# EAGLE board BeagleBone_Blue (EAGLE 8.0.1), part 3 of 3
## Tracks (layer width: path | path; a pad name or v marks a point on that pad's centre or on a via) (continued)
UART5_RX  (via drill 0.25 pad 0.46)
  Top 0.152: v68.38,34.29 68.73,34.29 69.01,34.57 70.46,34.57 71.04,33.98 71.04,26.36 70.31,25.63 68.15,25.63 67.06,24.54 67.06,22 67.51,21.54 69.42,21.54 v69.7,21.26 | 73.03,8.87 UT5.3 73,10.13 72.69,10.44 v69.7,10.44 | SIP.U2 62.31,37.52 v62.03,37.52
  Bottom 0.152: R131.2 63.32,32.51 63.5,32.69 65.48,32.69 65.84,33.05 65.84,34.24 | 65.84,34.49 65.35,34.98 64.06,34.98 63.88,35.15 63.88,35.94 63.7,36.12 62.99,36.12 62.79,36.32 62.79,37.03 62.31,37.52 v62.03,37.52 | 65.84,34.49 66.09,34.49 | 66.09,34.49 67.84,34.49 68.05,34.29 v68.38,34.29 | 65.84,34.49 65.84,34.24 | v69.7,21.26 v69.7,10.44 | 65.84,34.24 66.09,34.49
UART5_TX  (via drill 0.25 pad 0.46)
  Top 0.152: SIP.U1 63.42,36.75 62.97,36.75 62.76,36.55 62.31,36.55 v62.03,36.83 | v65.89,16.41 66.19,16.41 66.85,15.75 66.85,12.95 68.12,11.68 68.12,11.12 69.29,9.96 71.81,9.96 72.01,9.75 UT5.4
  Bottom 0.152: v65.89,16.41 66.06,16.59 66.06,20.22 65.05,21.23 65.05,22.63 56.01,31.67 53.29,31.67 51.77,33.2 51.77,33.68 52.05,33.96 56.9,33.96 58.73,35.79 59.64,35.79 60.07,35.36 60.07,35.1 60.35,34.82 60.86,34.82 61.21,35.18 61.21,35.59 60.27,36.52 60.27,36.93 60.55,37.21 61.65,37.21 v62.03,36.83 62.48,36.37 62.48,36.14 62.94,35.69 63.2,35.69 R129.2
USB0_D_N  (via drill 0.25 pad 0.46)
  Top 0.152: U3.2 8.03,39.57 7.49,39.04 6.88,39.04 6.48,38.63 v6.48,38.48 6.88,38.08 7.39,38.08 9.22,39.9 v9.73,39.9 | SIP.N18 41.96,31.8 v41.68,31.8
  Route2 0.152: v41.68,31.8 40.89,31.8 40.51,31.42 31.93,31.42 29.87,33.48 29.87,35.43 28.88,36.42 v27.79,36.42
  Bottom 0.152: X4.D- 5.7,37.7 v6.48,38.48 | v9.73,39.9 11.25,41.43 24.59,41.43 25.09,40.92 25.09,39.34 25.27,39.17 25.53,39.17 25.7,39.34 25.7,39.7 25.88,39.88 26.14,39.88 26.34,39.67 26.34,37.29 27.2,36.42 v27.79,36.42
USB0_D_P  (via drill 0.25 pad 0.46)
  Top 0.152: U3.1 7.53,39.58 7.29,39.34 6.76,39.34 6.4,38.99 6.17,38.99 v5.69,38.51 6.43,37.77 7.54,37.77 9.07,39.29 v9.3,39.29 | SIP.N17 43.16,32.13 42.67,31.65 42.32,31.65 41.81,31.14 v41.68,31.14
  Route2 0.152: v41.68,31.14 41.66,31.11 31.8,31.11 29.57,33.35 29.57,35.08 28.88,35.76 v27.79,35.76
  Bottom 0.152: X4.D+ 5.54,38.35 v5.69,38.51 | v9.3,39.29 9.96,39.29 11.79,41.12 24.43,41.12 24.77,40.79 24.77,39.06 24.97,38.86 25.58,38.86 26.04,38.41 26.04,37.13 27.41,35.76 v27.79,35.76
USB0_ID  (via drill 0.25 pad 0.46)
  Top 0.152: v7.19,38.56 7.44,38.56 8.53,39.64 U3.3 8.79,39.96 9.45,40.62 v9.7,40.62 | SIP.P16 44.35,32.92 41.88,32.92 v41.68,33.12
  Route2 0.152: v41.68,33.12 41.35,33.12 40.26,32.03 32.18,32.03 30.48,33.73 30.48,35.69 28.27,37.9 28.27,37.97 28.02,38.23 27.58,38.23 27.3,37.95 27.3,37.31 27.53,37.08 v27.79,37.08
  Bottom 0.152: X4.ID 6.74,39 v7.19,38.56 | v27.79,37.08 27.23,37.08 26.64,37.67 26.64,39.83 24.74,41.73 10.82,41.73 v9.7,40.62
USB0_VBUS  (via drill 0.25 pad 0.46)
  Top 0.152: v6.93,39.83 7.11,40 7.11,40.56 7.26,40.71 U3.6 7.53,41.63 R149.2 C54.1
  Bottom 0.152: v6.93,39.83 7.42,39.83 7.75,39.5 7.75,37.97 7.57,37.8 6.96,37.8 6.77,37.61 R112.2
  pour Bottom (no thermals): 3.45,37.21 5.99,37.21 6.2,37.41 7.32,37.41 7.32,36.55 6.2,36.55 5.89,36.86 3.45,36.86
USB1_D_N  (via drill 0.25 pad 0.46)
  Top 0.152: SIP.R18 42.29,34.21 v42.93,33.58 | v31.04,21.08 28.65,18.69 28.65,17.02 27.74,16.1 20.47,16.1 19.94,15.57 19.94,11.41 19.18,10.64 13.99,10.64 v13.74,10.39
  Bottom 0.152: v42.93,33.58 43.08,33.58 44.83,31.83 44.83,31.22 45.26,30.79 45.49,30.79 47.68,28.6 47.68,26.8 46.53,25.65 37.03,25.65 32.94,21.56 31.52,21.56 v31.04,21.08 | v13.74,10.39 13.34,9.98 13.34,9.4 13.13,9.2 12.9,9.2 12.72,9.37 12.72,9.73 12.52,9.93 12.24,9.93 12.06,9.75 12.06,9.4 11.89,9.22 11.25,9.22 X3.2
  Bottom 0.254: X3.2 9.93,10.54 3.43,10.54 2.92,10.03 2.92,9.27 3.17,9.02 U4.2
USB1_D_P  (via drill 0.25 pad 0.46)
  Top 0.152: 43.56,34.62 43.23,34.29 v42.95,34.29 | v14.61,9.98 14.96,10.34 19.3,10.34 20.24,11.28 20.24,15.44 20.6,15.8 27.86,15.8 28.96,16.89 28.96,18.57 30.96,20.57 31.24,20.57 v31.75,21.08
  Top 0.254: SIP.R17 43.56,34.62
  Bottom 0.152: v42.95,34.29 43.26,34.29 43.71,33.83 43.71,33.38 45.16,31.93 45.16,31.32 45.39,31.09 45.62,31.09 47.98,28.73 47.98,26.67 46.66,25.35 37.16,25.35 32.89,21.08 v31.75,21.08 | X3.3 13.53,8.02 14.61,9.09 v14.61,9.98
  Bottom 0.254: U4.1 3.18,8.52 2.92,8.26 2.92,7.62 3.3,7.24 9.54,7.24 10.32,8.02 X3.3
USB1_VBUS  (via drill 0.25 pad 0.46)
  Top 0.254: v11.43,11.3 8.89,11.3 7.87,10.29 7.87,9.02 6.99,8.13 v6.48,8.13
  Bottom 0.254: U4.6 5.53,8.52 C55.1 6.15,8.46 v6.48,8.13 | v11.43,11.3 16.26,11.3 C45.1
  pour Bottom (no thermals): 15.85,12.98 20.95,12.98 20.95,13.72 22.48,13.72 22.48,12.19 20.32,12.19 20.32,10.29 19.18,10.29 19.18,10.67 17.14,10.67 17.14,10.97 15.85,10.97
USB_DC  (via drill 0.81)
  Bottom 0.813: R112.1 8.47,41.72 9.42,42.67 25.3,42.67 27.2,40.77 37.13,40.77 38.71,42.34 47.3,42.34 47.73,41.91 v54.36,41.91 54.38,41.91
  pour Top: 53.09,41.91 53.09,40.67 53.34,40.41 53.72,40.41 53.72,41.02 54.99,41.02 54.99,40.41 55.37,40.41 55.63,40.67 55.63,41.91 54.74,42.8 53.98,42.8
USR_LED0  (via drill 0.25 pad 0.46)
  Top 0.152: SIP.V15 46.89,37.69 46.89,37.01 47.04,36.86 v47.04,36.58 | v26.16,5.46 25.63,5.46 25.4,5.69 0.A
  Bottom 0.152: 47.04,36.37 v47.04,36.58 47.04,36.3 47.9,35.43 47.9,35.08 48.54,34.44 48.54,34.21 49.76,33 49.76,32.79 50.16,32.38 50.42,32.38 52.65,30.15 55.32,30.15 63.52,21.95 63.52,20.19 63.7,20.02 63.7,6.17 62.28,4.75 26.87,4.75 v26.16,5.46
USR_LED1  (via drill 0.25 pad 0.46)
  Top 0.152: SIP.U15 46.38,36.93 v46.38,36.58 | v27.69,5.49 27.15,5.49 26.92,5.71 1.A
  Bottom 0.152: 46.38,36.5 v46.38,36.58 46.38,36.47 47.6,35.25 47.6,34.95 48.23,34.31 48.23,34.09 49.45,32.87 49.45,32.66 50.04,32.08 50.29,32.08 52.55,29.82 55.22,29.82 63.22,21.82 63.22,20.07 63.4,19.89 63.4,6.3 62.15,5.05 28.12,5.05 v27.69,5.49
USR_LED2  (via drill 0.25 pad 0.46)
  Top 0.152: SIP.T15 46.71,35.33 v46.71,35.03 | v30.94,6.2 30.94,6.86 30.71,7.09 28.57,7.09 28.45,6.96 2.A
  Bottom 0.152: v46.71,35.03 46.97,34.77 46.97,33.78 47.42,33.33 47.7,33.33 48.54,32.49 48.54,32.28 49.66,31.17 49.91,31.17 52.17,28.91 54.84,28.91 62.08,21.67 62.08,18.44 62.79,17.73 62.79,6.55 61.9,5.66 31.77,5.66 31.24,6.2 v30.94,6.2
USR_LED3  (via drill 0.25 pad 0.46)
  Top 0.152: SIP.V16 45.62,37.69 45.62,37.01 45.72,36.91 v45.72,36.58 | v30.94,5.54 30.15,5.54 29.97,5.71 3.A
  Bottom 0.152: v45.72,36.58 45.72,36.45 46.08,36.09 46.33,36.09 47.27,35.15 47.27,33.91 47.55,33.63 47.83,33.63 48.84,32.61 48.84,32.41 49.78,31.47 50.04,31.47 52.3,29.21 54.97,29.21 62.38,21.79 62.38,18.57 63.09,17.86 63.09,6.43 62.03,5.36 31.11,5.36 v30.94,5.54
V_BATT  (via drill 0.25 pad 0.46, 0.5)
  Top 0.254: CHGIC.9 24.64,48.01 v26.42,46.23
  Top 0.406: H2.13 85.16,28.64 v84.71,28.19 | H2.14 84.51,29.01 v83.69,28.19 | H1.24 70.11,11.56 v70.61,12.06 | H1.13 70.15,18.71 v70.74,19.3 | H1.14 v70.73,18.06 v70.74,18.06 | H2.24 78.01,28.71 v77.5,28.19
  Bottom 0.152: R19.1 70.64,9.78
  Bottom 0.254: R34.1 R28.1 27.13,46.23 v26.42,46.23 26.42,47.62 27.69,48.89 R4.1
  other vias: 51.05,49.66 51.05,48.77 51.94,48.77 51.94,49.66 70.48,24.64 71.37,24.64 69.6,24.64
  pour Bottom (rank 2, no thermals): 26.92,50.55 28.83,50.55 28.83,50.67 32.26,50.67 32.26,49.48 38.66,49.48 38.66,52.58 42.42,52.58 42.42,49.91 50.67,49.91 50.67,51.05 52.32,51.05 52.32,48.39 50.67,48.39 50.67,49.02 41.66,49.02 41.66,50.04 39.5,50.04 39.5,48.51 26.92,48.51
  pour Top (no thermals): 39.62,50.55 39.62,52.45 44.83,52.45 44.83,52.32 44.83,50.29 39.62,50.29
  pour Top (no thermals): 57.53,50.67 57.53,47.88 53.72,47.88 53.72,48.39 50.67,48.39 50.67,50.04 53.72,50.04 53.72,50.67
  pour Route2 (isolate 0.254, rank 5, no thermals): 50.67,50.04 77.47,50.04 77.47,24 69.09,24 69.09,25.27 75.82,25.27 75.82,48.39 50.67,48.39
  pour Top: 68.45,21.97 68.45,25.27 72.39,25.27 72.39,21.97
  pour Bottom: 68.83,25.27 76.45,25.27 76.45,28.7 85.22,28.7 85.22,24 75.18,24 75.18,9.27 70.23,9.27 70.23,22.35 68.83,22.35
V_DIV_BAT  (via drill 0.25 pad 0.46)
  Top 0.152: SIP.A8 54.99,16.48 56.39,15.09 58.45,15.09 58.75,14.78 58.75,12.75 59.31,12.19 65.86,12.19 v65.96,12.29
  Bottom 0.152: R25.1 R19.2 66.95,9.78 66.85,9.88 66.85,11.91 66.47,12.29 v65.96,12.29
V_DIV_DC  (via drill 0.25 pad 0.46)
  Top 0.152: v55.63,16.71 55.63,17.53 SIP.B8
  Bottom 0.152: R1.2 R14.1 58.73,15.6 58.52,15.8 56.54,15.8 v55.63,16.71
VCC  (via drill 0.25 pad 0.46, 0.5)
  Top 0.152: CHG.A 36.33,44.45 36.96,44.45 40.13,47.62 41.78,47.62 | v66.04,6.68 64.44,6.68 61.01,10.11 v61.01,10.57 | 41.78,47.62 41.91,47.5 | 42.04,47.37 42.29,47.12 v42.75,47.12 | v42.42,48.26 42.04,47.88 | 42.04,47.88 41.91,47.75 | 41.91,47.75 41.78,47.62 | 42.04,47.88 42.04,47.37 | 42.04,47.37 41.91,47.5 | 41.91,47.5 41.91,47.75
  Top 0.254: CHGIC.2 17.65,48.51
  Top 0.61: v42.42,48.26 43.31,49.15 45.09,49.15 45.82,49.89 45.82,50.91 D3.A
  Route2 0.152: v76.07,10.13 76.07,9.68 76.58,9.17 77.52,9.17 77.8,9.45 77.8,9.83 78.69,10.72 78.69,15.27 79.6,16.18 80.42,16.18 81.03,15.57 81.79,15.57 82.17,15.95 82.17,16.28 83.06,17.17 83.06,29.87 84.35,31.17 84.35,32.97 v84.15,33.17
  Route2 0.61: v17.2,47.88 24.89,47.88 25.65,47.12 38.86,47.12 39.42,47.68 41.83,47.68 v42.42,48.26
  Bottom 0.152: v76.07,10.13 76.07,9.73 75.59,9.25 72.67,9.25 70.1,6.68 v66.04,6.68 | v61.01,10.57 61.01,12.17 59.89,13.28 R1.1 | v42.75,47.12 43.71,46.15 43.71,44.55 44.07,44.2 47.17,44.2 47.7,44.73 49.66,44.73 50.22,45.29 51.82,45.29 52.43,45.9 52.43,46.58 53.24,47.4 53.24,47.9 52.68,48.46 52.68,51.54 52.48,51.74 52.48,52.22 52.78,52.53 53.16,52.53 53.49,52.2 53.49,51.74 53.29,51.54 53.29,50.57 53.44,50.42 56.26,50.42 56.92,49.76 74.85,49.76 84.33,40.28 84.33,33.35 v84.15,33.17
  pour Top: 9.02,52.45 9.02,45.97 17.65,45.97 17.65,48.51 12.19,48.51 12.19,52.45
VCC_CHG
  Top 0.254: CHGIC.3 20.07,48.01 19.81,47.75 R5.2 C4.2
VDD_1V8  (via drill 0.25 pad 0.46, 0.5)
  Top 0.254: C47.1 7.34,22.07 7.07,21.8 OSC1.4 7.19,21.16 R90.2 | U10.2 v21.52,31.54 v21.51,31.55 | v21.51,32.61 21.82,32.92 C50.1 v21.82,40.28 22.39,40.86 U2.5 | R105.1 19.66,42.72 20.7,41.68 v20.7,40.28 | SIP.R16 44.83,34.24 v45.03,34.04 | SIP.N16 45.39,31.57 v45.64,31.57 | 9.42,19.94 9.39,19.9
  Top 0.406: R9.1 R102.1 R101.1 R99.1 R98.1 R103.1 R105.1 | U7.38 9.23,24.05 9.6,23.67 C57.2 C47.1 9.6,21.41 v9.42,21.23 9.42,19.94 | 9.39,19.9 C60.2
  Route2 0.61: v37.77,21.67 40.34,21.67 41.27,22.61 47.85,22.61 48.44,23.19 48.44,24.31 v49.28,25.15 v53.09,21.34 | v9.42,21.23 20.04,21.23 20.8,20.47 v29.11,20.47
  Bottom 0.254: v21.51,31.55 18.21,31.55 17.7,31.04 | v21.51,32.61 18.03,32.61 17.7,32.28 | v20.7,40.28 20.4,39.98 C52.1 20.88,39.34 v21.82,40.28 | v49.28,25.15 49.28,27.94 v45.64,31.57 45.64,32.18 45.39,32.44 45.39,33.68 v45.03,34.04
  Bottom 0.305: v9.42,21.23 9.42,21.87 12.62,25.07 16.79,25.07 17.7,25.98 17.7,31.04 17.7,32.28 17.7,33.17 18.34,33.81 U9.2
  Bottom 0.61: v37.77,21.67 37.29,21.18 34.14,21.18 33.33,20.37 29.21,20.37 v29.11,20.47
  pour Top: 52.45,20.7 52.45,21.97 53.72,21.97 53.72,20.7
VDD_3V3AUX
  Top 0.152: SIP.Y11 50.62,41.58 48.69,41.58 47.68,42.6 35.66,42.6 34.82,41.76 29.62,41.76 28.27,43.1 21.84,43.1 21.16,43.79 17.17,43.79 16.76,44.2 13.46,44.2 13.2,44.46 ON.A
VDD_ADC  (via drill 0.25 pad 0.46)
  Top 0.152: SIP.D8 54.99,20.32 v55.24,20.07 55.63,20.07 55.78,19.91 56.49,19.91 56.74,19.66 56.74,19.1 57.2,18.64 57.81,18.64 58.01,18.44 58.01,18.11 58.8,17.32 SIP.A5 59.26,16.89 v59.44,17.07 59.61,16.89 SIP.A4 60.07,16.26 61.49,14.83 61.77,14.83 62.03,14.58 63.32,14.58 63.69,14.21 ADC.2
  Bottom 0.152: R111.1 58.98,17.53 v59.44,17.07 | C44.1 55.5,20.95 55.24,20.7 v55.24,20.07
VDD_RTC  (via drill 0.25 pad 0.46)
  Top 0.152: SIP.E14 47.8,21.54 v47.8,21.34 | v40.41,14.66 39.16,13.4 U6.5
  Bottom 0.152: v47.8,21.34 47.32,21.82 46.15,21.82 45.95,21.62 45.95,20.02 46.74,19.23 47.35,19.23 48.31,18.26 48.31,16.51 46.81,15.01 41.48,15.01 41.12,14.66 v40.41,14.66
WIFI_LED  (via drill 0.25 pad 0.46)
  Top 0.152: WIFI.A 27.99,22.73 28.78,21.95 32.56,21.95 32.99,21.51 35.51,21.51 36.68,20.34 v36.68,17.58 | SIP.A15 46.53,16.89 v46.74,17.09
  Bottom 0.152: v36.68,17.58 37.62,16.64 38.46,16.64 41.12,19.3 43.05,19.3 43.56,19.81 44.3,19.81 44.73,19.38 44.73,18.14 45.34,17.53 46.23,17.53 46.66,17.09 v46.74,17.09
WL_BT_OE  (via drill 0.25 pad 0.46)
  Top 0.152: SIP.L18 42.29,30.15 41.96,30.48 v41.68,30.48 | R93.1 24.46,36.45 v25.38,37.36
  Bottom 0.152: v41.68,30.48 41.27,30.07 36.42,30.07 35.66,29.31 31.76,29.31 29.37,31.7 27.58,31.7 27.36,31.93 27.36,35.38 v25.38,37.36
WL_EN  (via drill 0.25 pad 0.46)
  Top 0.152: SIP.K18 42.29,28.83 42.14,28.98 v41.66,28.98 | v27.13,30.35 26.8,30.35 26.54,30.61 26.54,31.27 26.77,31.5 27.33,31.5 27.43,31.39 28.27,31.39 28.63,31.75 28.63,34.42 28.37,34.67 27.38,34.67 27.05,34.34 27.05,33.38 26.77,33.1 25.81,33.1 25.38,32.66 v24.23,32.66
  Bottom 0.152: U9.20 22.6,33.33 23.57,33.33 v24.23,32.66 | v41.66,28.98 41.45,28.78 36.42,28.78 36.04,28.4 31.19,28.4 29.06,30.53 27.3,30.53 v27.13,30.35
WL_EN_1V8  (via drill 0.25 pad 0.46)
  Top 0.152: U7.40 10.62,24.55 | 10.63,24.09 U7.40 | U7.40 10.63,24.09 11.1,23.62 11.56,23.62 v11.79,23.39 12.57,22.61 R87.1
  Bottom 0.152: v11.79,23.39 13.08,24.69 17.02,24.69 18.09,25.76 18.09,29.92 19.1,30.94 21.87,30.94 22.12,31.19 22.12,33 21.78,33.34 U9.1
WL_IRQ  (via drill 0.25 pad 0.46)
  Top 0.152: R84.1 11.46,40.44 11.63,40.26 v11.63,39.83 | v23.34,40.39 U2.2
  Bottom 0.152: v11.63,39.83 12.62,40.82 22.91,40.82 v23.34,40.39
WL_SDIO_CLK  (via drill 0.25 pad 0.46)
  Top 0.152: R103.2 R78.1 18.36,40.44 18.62,40.18 v18.62,38.48
  Bottom 0.152: v18.62,38.48 18.62,37.97 18.62,37.69 19.5,36.81 U9.8
WL_SDIO_CMD  (via drill 0.25 pad 0.46)
  Top 0.152: R105.2 R79.1 19.68,40.44 19.89,40.23 v19.89,38.28
  Bottom 0.152: v19.89,38.28 20.12,38.05 U9.9
WL_SDIO_D0  (via drill 0.25 pad 0.46)
  Top 0.152: R98.2 R80.1 17.02,40.44 17.25,40.21 v17.25,38.58
  Bottom 0.152: v17.25,38.58 19.52,36.31 U9.7
WL_SDIO_D1  (via drill 0.25 pad 0.46)
  Top 0.152: R99.2 R81.1 15.65,40.44 15.85,40.23 v15.85,38.91
  Bottom 0.152: v15.85,38.91 15.85,38.66 16.43,38.08 17.17,38.08 19.43,35.81 U9.6
WL_SDIO_D2  (via drill 0.25 pad 0.46)
  Top 0.152: R101.2 R82.1 14.22,40.44 14.43,40.23 v14.43,39.19
  Bottom 0.152: v14.43,39.19 14.86,39.19 16.28,37.77 16.89,37.77 19.35,35.31 U9.5
WL_SDIO_D3  (via drill 0.25 pad 0.46)
  Top 0.152: R102.2 R83.1 12.88,40.44 13.06,40.26 v13.06,39.78
  Bottom 0.152: v13.06,39.78 14.15,38.68 14.91,38.68 16.13,37.47 16.71,37.47 19.37,34.81 U9.4
WLAN_IRQ  (via drill 0.25 pad 0.46)
  Top 0.152: SIP.K16 44.58,28.32 v44.2,28.7 | v27.08,31.01 28.32,31.01 28.93,31.62 28.93,34.57 28.52,34.98 27.66,34.98 27.3,35.33 27.3,38.15 26.72,38.73 26.72,41.05 25.88,41.89 U2.4
  Bottom 0.152: v44.2,28.7 43.43,29.46 41.02,29.46 40.64,29.08 36.3,29.08 35.92,28.7 31.32,28.7 29.18,30.84 27.25,30.84 v27.08,31.01

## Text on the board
Bottom: jw | e
tPlace: J2 | 8 | 3 | 4 | 7 | 6 | 5 | 4 | 3 | 2 | 2 | 1 | 1 | 3 | 4 | 2 | 1
bPlace: BAL | BeagleBone Blue / Rev A2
